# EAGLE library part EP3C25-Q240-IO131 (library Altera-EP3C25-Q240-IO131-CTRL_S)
EPF10K30 FLEX 10K family
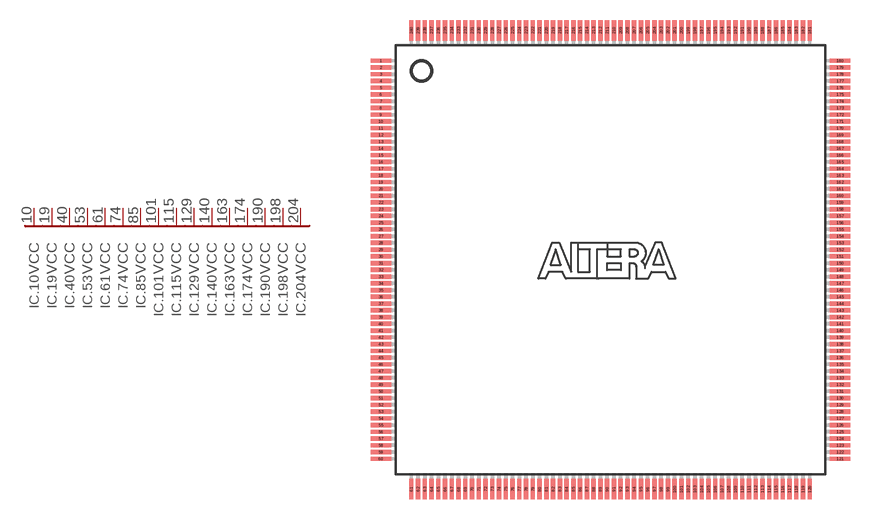
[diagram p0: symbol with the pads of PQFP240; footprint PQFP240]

Designator prefix IC; gates .10=VCCINT .19=VCCINT .40=VCCINT .53=VCCINT .61=VCCINT .74=VCCINT .85=VCCINT .101=VCCINT .115=VCCINT .129=VCCINT .140=VCCINT .163=VCCINT .174=VCCINT .190=VCCINT .198=VCCINT .204=VCCINT .222=VCCINT .228=VCCINT -8=GNDINT -11=GNDINT -16=GNDINT -20=GNDINT -36=GNDINT -42=GNDINT -48=GNDINT -54=GNDINT -62=GNDINT -67=GNDINT -75=GNDINT -79=GNDINT -86=GNDINT -97=GNDINT -102=GNDINT -105=GNDINT -116=GNDINT -125=GNDINT -130=GNDINT -138=GNDINT -141=GNDINT -156=GNDINT -165=GNDINT -175=GNDINT -191=GNDINT -193=GNDINT -199=GNDINT -205=GNDINT -208=GNDINT -215=GNDINT -222=GNDINT -227=GNDINT -229=GNDINT -172=GNDINT _B1_V=VCC_IO _B2_V=VCC_IO _B3_V=VCC_IO _B4_V=VCC_IO _B5_V=VCC_IO _B6_V=VCC_IO _B7_V=VCC_IO _B8_V=VCC_IO -IO=IO_1-131 _IO=INFO-BUS _CRTL=INFO-BUS G$2=USAGE G$31=CONF_DONE PLL1=VCCD PLL2=VCCD PLL3=VCCD PLL4=VCCD GNDA1=GNDA GNDA2=GNDA GNDA3=GNDA GNDA4=GNDA VCCA1=VCCA VCCA2=VCCA VCCA3=VCCA VCCA4=VCCA _CLK0=CLK _CLK1=CLK _CLK2=CLK _CLK3=CLK _CLK4=CLK _CLK5=CLK _CLK6=CLK _CLK7=CLK _CLK8=CLK _CLK9=CLK _CLK10=CLK _CLK11=CLK _CLK12=CLK _CLK13=CLK _CLK14=CLK _CLK15=CLK _MSEL0=MSEL _MSEL1=MSEL _MSEL2=MSEL _/CE=CTRL _/CONFIG=CTRL _/STATUS=CTRL _TCK=JTAG-IN _TMS=JTAG-IN _TDI=JTAG-IN _TDO=JTAG-OUT _DCLK=CTRL _DATA0=CTRL

## EP3C25-Q240-IO131 (BUS-CTRL: -CTRL:CLK[0..15],CONF_DONE,/STATUS,/CONFIG,MSEL[0..2],/CE,DCLK,DATA0,TCK,TDO,TMS,TDI; BUS-IO: -IO:PIN#,4,5,6,9,12,13,14,18,21,22,37,38,39,41,42,43,44,45,46,49,50,51,52,55,56,57,63,64,65,68,69,70,71,72,73,76,78,80,81,82,83,84,87,88,93,94,95,98,99,100,103,106,107,108,109,110,111,112,113,114,117,118,119,120,126,127,128,131,132,133,134,135,137,139,142,148,159,160,161,162,164,166,167,168,169,171,173,176,177,181,182,183,184,185,186,187,188,189,194,195,196,197,200,201,202,203,207,214,216,217,218,219,221,223,224,226,230,231,232,233,234,235,236,237,238,239,240)  [PQFP240]
1  PLL3:VCCD  pwr
2  GNDA3:GNDA  pwr
3  VCCA3:VCCA  pwr
4  -IO:IO_1
5  -IO:IO_2
6  -IO:IO_3
7  _B1_V:VCC1  pwr
8  -8:GND  pwr
9  -IO:IO_4
10  .10:VCC  pwr
11  -11:GND  pwr
12  -IO:IO_5
13  -IO:IO_6
14  -IO:IO_7
15  _B1_V:VCC2  pwr
16  -16:GND  pwr
17  _/STATUS:P$1  in
18  -IO:IO_8
19  .19:VCC  pwr
20  -20:GND  pwr
21  -IO:IO_9
22  -IO:IO_10
23  _DCLK:P$1  in
24  _DATA0:P$1  in
25  _/CONFIG:P$1  in
26  _TDI:P$1  in
27  _TCK:P$1  in
28  _TMS:P$1  in
29  _TDO:P$1  out
30  _/CE:P$1  in
31  _CLK0:CLK  out
32  _CLK1:CLK  out
33  _CLK2:CLK  out
34  _CLK3:CLK  out
35  _B2_V:VCC1  pwr
36  -36:GND  pwr
37  -IO:IO_11
38  -IO:IO_12
39  -IO:IO_13
40  .40:VCC  pwr
41  -IO:IO_14
42  -42:GND  pwr
43  -IO:IO_15
44  -IO:IO_16
45  -IO:IO_17
46  -IO:IO_18
47  _B2_V:VCC2  pwr
48  -48:GND  pwr
49  -IO:IO_19
50  -IO:IO_20
51  -IO:IO_21
52  -IO:IO_22
53  .53:VCC  pwr
54  -54:GND  pwr
55  -IO:IO_23
56  -IO:IO_24
57  -IO:IO_25
58  VCCA1:VCCA  pwr
59  GNDA1:GNDA  pwr
60  PLL1:VCCD  pwr
61  .61:VCC  pwr
62  -62:GND  pwr
63  -IO:IO_26
64  -IO:IO_27
65  -IO:IO_28
66  _B3_V:VCC1  pwr
67  -67:GND  pwr
68  -IO:IO_29
69  -IO:IO_30
70  -IO:IO_31
71  -IO:IO_32
72  -IO:IO_33
73  -IO:IO_34
74  .74:VCC  pwr
75  -75:GND  pwr
76  -IO:IO_35
77  _B3_V:VCC2  pwr
78  -IO:IO_36
79  -79:GND  pwr
80  -IO:IO_37
81  -IO:IO_38
82  -IO:IO_39
83  -IO:IO_40
84  -IO:IO_41
85  .85:VCC  pwr
86  -86:GND  pwr
87  -IO:IO_42
88  -IO:IO_43
89  _CLK15:CLK  out
90  _CLK14:CLK  out
91  _CLK13:CLK  out
92  _CLK12:CLK  out
93  -IO:IO_44
94  -IO:IO_45
95  -IO:IO_46
96  _B4_V:VCC1  pwr
97  -97:GND  pwr
98  -IO:IO_47
99  -IO:IO_48
100  -IO:IO_49
101  .101:VCC  pwr
102  -102:GND  pwr
103  -IO:IO_50
104  _B4_V:VCC2  pwr
105  -105:GND  pwr
106  -IO:IO_51
107  -IO:IO_52
108  -IO:IO_53
109  -IO:IO_54
110  -IO:IO_55
111  -IO:IO_56
112  -IO:IO_57
113  -IO:IO_58
114  -IO:IO_59
115  .115:VCC  pwr
116  -116:GND  pwr
117  -IO:IO_60
118  -IO:IO_61
119  -IO:IO_62
120  -IO:IO_63
121  PLL4:VCCD  pwr
122  GNDA4:GNDA  pwr
123  VCCA4:VCCA  pwr
124  _B5_V:VCC1  pwr
125  -125:GND  pwr
126  -IO:IO_64
127  -IO:IO_65
128  -IO:IO_66
129  .129:VCC  pwr
130  -130:GND  pwr
131  -IO:IO_67
132  -IO:IO_68
133  -IO:IO_69
134  -IO:IO_70
135  -IO:IO_71
136  _B5_V:VCC2  pwr
137  -IO:IO_72
138  -138:GND  pwr
139  -IO:IO_73
140  .140:VCC  pwr
141  -141:GND  pwr
142  -IO:IO_74
143  -IO:IO_75
144  -IO:IO_76
145  -IO:IO_77
146  -IO:IO_78
147  -IO:IO_79
148  -IO:IO_80
149  _CLK7:CLK  out
150  _CLK6:CLK  out
151  _CLK5:CLK  out
152  _CLK4:CLK  out
153  G$31:CONF_DONE  out
154  _B6_V:VCC1  pwr
155  _MSEL0:MSEL  in
156  -156:GND  pwr
157  _MSEL1:MSEL  in
158  _MSEL2:MSEL  in
159  -IO:IO_81
160  -IO:IO_82
161  -IO:IO_83
162  -IO:IO_84
163  .163:VCC  pwr
164  -IO:IO_85
165  -165:GND  pwr
166  -IO:IO_86
167  -IO:IO_87
168  -IO:IO_88
169  -IO:IO_89
170  _B6_V:VCC2  pwr
171  -IO:IO_90
172  -172:GND  pwr
173  -IO:IO_91
174  .174:VCC  pwr
175  -175:GND  pwr
176  -IO:IO_92
177  -IO:IO_93
178  VCCA2:VCCA  pwr
179  GNDA2:GNDA  pwr
180  PLL2:VCCD  pwr
181  -IO:IO_94
182  -IO:IO_95
183  -IO:IO_96
184  -IO:IO_97
185  -IO:IO_98
186  -IO:IO_99
187  -IO:IO_100
188  -IO:IO_101
189  -IO:IO_102
190  .190:VCC  pwr
191  -191:GND  pwr
192  _B7_V:VCC1  pwr
193  -193:GND  pwr
194  -IO:IO_103
195  -IO:IO_104
196  -IO:IO_105
197  -IO:IO_106
198  .198:VCC  pwr
199  -199:GND  pwr
200  -IO:IO_107
201  -IO:IO_108
202  -IO:IO_109
203  -IO:IO_110
204  .204:VCC  pwr
205  -205:GND  pwr
206  _B7_V:VCC2  pwr
207  -IO:IO_111
208  -208:GND  pwr
209  _CLK8:CLK  out
210  _CLK9:CLK  out
211  _CLK10:CLK  out
212  _CLK11:CLK  out
213  _B8_V:VCC1  pwr
214  -IO:IO_112
215  -215:GND  pwr
216  -IO:IO_113
217  -IO:IO_114
218  -IO:IO_115
219  -IO:IO_116
220  .222:VCC  pwr
221  -IO:IO_117
222  -222:GND  pwr
223  -IO:IO_118
224  -IO:IO_119
225  _B8_V:VCC2  pwr
226  -IO:IO_120
227  -227:GND  pwr
228  .228:VCC  pwr
229  -229:GND  pwr
230  -IO:IO_121
231  -IO:IO_122
232  -IO:IO_123
233  -IO:IO_124
234  -IO:IO_125
235  -IO:IO_126
236  -IO:IO_127
237  -IO:IO_128
238  -IO:IO_129
239  -IO:IO_130
240  -IO:IO_131

## Footprint PQFP240 (pad centres in mm)
Plastic Quad Flat Pack
smd 1.5 x 0.32: 1 -17,14.75; 2 -17,14.25; 3 -17,13.75; 4 -17,13.25; 5 -17,12.75; 6 -17,12.25; 7 -17,11.75; 8 -17,11.25; 9 -17,10.75; 10 -17,10.25; 11 -17,9.75; 12 -17,9.25; 13 -17,8.75; 14 -17,8.25; 15 -17,7.75; 16 -17,7.25; 17 -17,6.75; 18 -17,6.25; 19 -17,5.75; 20 -17,5.25; 21 -17,4.75; 22 -17,4.25; 23 -17,3.75; 24 -17,3.25; 25 -17,2.75; 26 -17,2.25; 27 -17,1.75; 28 -17,1.25; 29 -17,0.75; 30 -17,0.25; 31 -17,-0.25; 32 -17,-0.75; 33 -17,-1.25; 34 -17,-1.75; 35 -17,-2.25; 36 -17,-2.75; 37 -17,-3.25; 38 -17,-3.75; 39 -17,-4.25; 40 -17,-4.75; 41 -17,-5.25; 42 -17,-5.75; 43 -17,-6.25; 44 -17,-6.75; 45 -17,-7.25; 46 -17,-7.75; 47 -17,-8.25; 48 -17,-8.75; 49 -17,-9.25; 50 -17,-9.75; 51 -17,-10.25; 52 -17,-10.75; 53 -17,-11.25; 54 -17,-11.75; 55 -17,-12.25; 56 -17,-12.75; 57 -17,-13.25; 58 -17,-13.75; 59 -17,-14.25; 60 -17,-14.75; 121 17,-14.75; 122 17,-14.25; 123 17,-13.75; 124 17,-13.25; 125 17,-12.75; 126 17,-12.25; 127 17,-11.75; 128 17,-11.25; 129 17,-10.75; 130 17,-10.25; 131 17,-9.75; 132 17,-9.25; 133 17,-8.75; 134 17,-8.25; 135 17,-7.75; 136 17,-7.25; 137 17,-6.75; 138 17,-6.25; 139 17,-5.75; 140 17,-5.25; 141 17,-4.75; 142 17,-4.25; 143 17,-3.75; 144 17,-3.25; 145 17,-2.75; 146 17,-2.25; 147 17,-1.75; 148 17,-1.25; 149 17,-0.75; 150 17,-0.25; 151 17,0.25; 152 17,0.75; 153 17,1.25; 154 17,1.75; 155 17,2.25; 156 17,2.75; 157 17,3.25; 158 17,3.75; 159 17,4.25; 160 17,4.75; 161 17,5.25; 162 17,5.75; 163 17,6.25; 164 17,6.75; 165 17,7.25; 166 17,7.75; 167 17,8.25; 168 17,8.75; 169 17,9.25; 170 17,9.75; 171 17,10.25; 172 17,10.75; 173 17,11.25; 174 17,11.75; 175 17,12.25; 176 17,12.75; 177 17,13.25; 178 17,13.75; 179 17,14.25; 180 17,14.75
smd 0.32 x 1.5: 61 -14.75,-17; 62 -14.25,-17; 63 -13.75,-17; 64 -13.25,-17; 65 -12.75,-17; 66 -12.25,-17; 67 -11.75,-17; 68 -11.25,-17; 69 -10.75,-17; 70 -10.25,-17; 71 -9.75,-17; 72 -9.25,-17; 73 -8.75,-17; 74 -8.25,-17; 75 -7.75,-17; 76 -7.25,-17; 77 -6.75,-17; 78 -6.25,-17; 79 -5.75,-17; 80 -5.25,-17; 81 -4.75,-17; 82 -4.25,-17; 83 -3.75,-17; 84 -3.25,-17; 85 -2.75,-17; 86 -2.25,-17; 87 -1.75,-17; 88 -1.25,-17; 89 -0.75,-17; 90 -0.25,-17; 91 0.25,-17; 92 0.75,-17; 93 1.25,-17; 94 1.75,-17; 95 2.25,-17; 96 2.75,-17; 97 3.25,-17; 98 3.75,-17; 99 4.25,-17; 100 4.75,-17; 101 5.25,-17; 102 5.75,-17; 103 6.25,-17; 104 6.75,-17; 105 7.25,-17; 106 7.75,-17; 107 8.25,-17; 108 8.75,-17; 109 9.25,-17; 110 9.75,-17; 111 10.25,-17; 112 10.75,-17; 113 11.25,-17; 114 11.75,-17; 115 12.25,-17; 116 12.75,-17; 117 13.25,-17; 118 13.75,-17; 119 14.25,-17; 120 14.75,-17; 181 14.75,17; 182 14.25,17; 183 13.75,17; 184 13.25,17; 185 12.75,17; 186 12.25,17; 187 11.75,17; 188 11.25,17; 189 10.75,17; 190 10.25,17; 191 9.75,17; 192 9.25,17; 193 8.75,17; 194 8.25,17; 195 7.75,17; 196 7.25,17; 197 6.75,17; 198 6.25,17; 199 5.75,17; 200 5.25,17; 201 4.75,17; 202 4.25,17; 203 3.75,17; 204 3.25,17; 205 2.75,17; 206 2.25,17; 207 1.75,17; 208 1.25,17; 209 0.75,17; 210 0.25,17; 211 -0.25,17; 212 -0.75,17; 213 -1.25,17; 214 -1.75,17; 215 -2.25,17; 216 -2.75,17; 217 -3.25,17; 218 -3.75,17; 219 -4.25,17; 220 -4.75,17; 221 -5.25,17; 222 -5.75,17; 223 -6.25,17; 224 -6.75,17; 225 -7.25,17; 226 -7.75,17; 227 -8.25,17; 228 -8.75,17; 229 -9.25,17; 230 -9.75,17; 231 -10.25,17; 232 -10.75,17; 233 -11.25,17; 234 -11.75,17; 235 -12.25,17; 236 -12.75,17; 237 -13.25,17; 238 -13.75,17; 239 -14.25,17; 240 -14.75,17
